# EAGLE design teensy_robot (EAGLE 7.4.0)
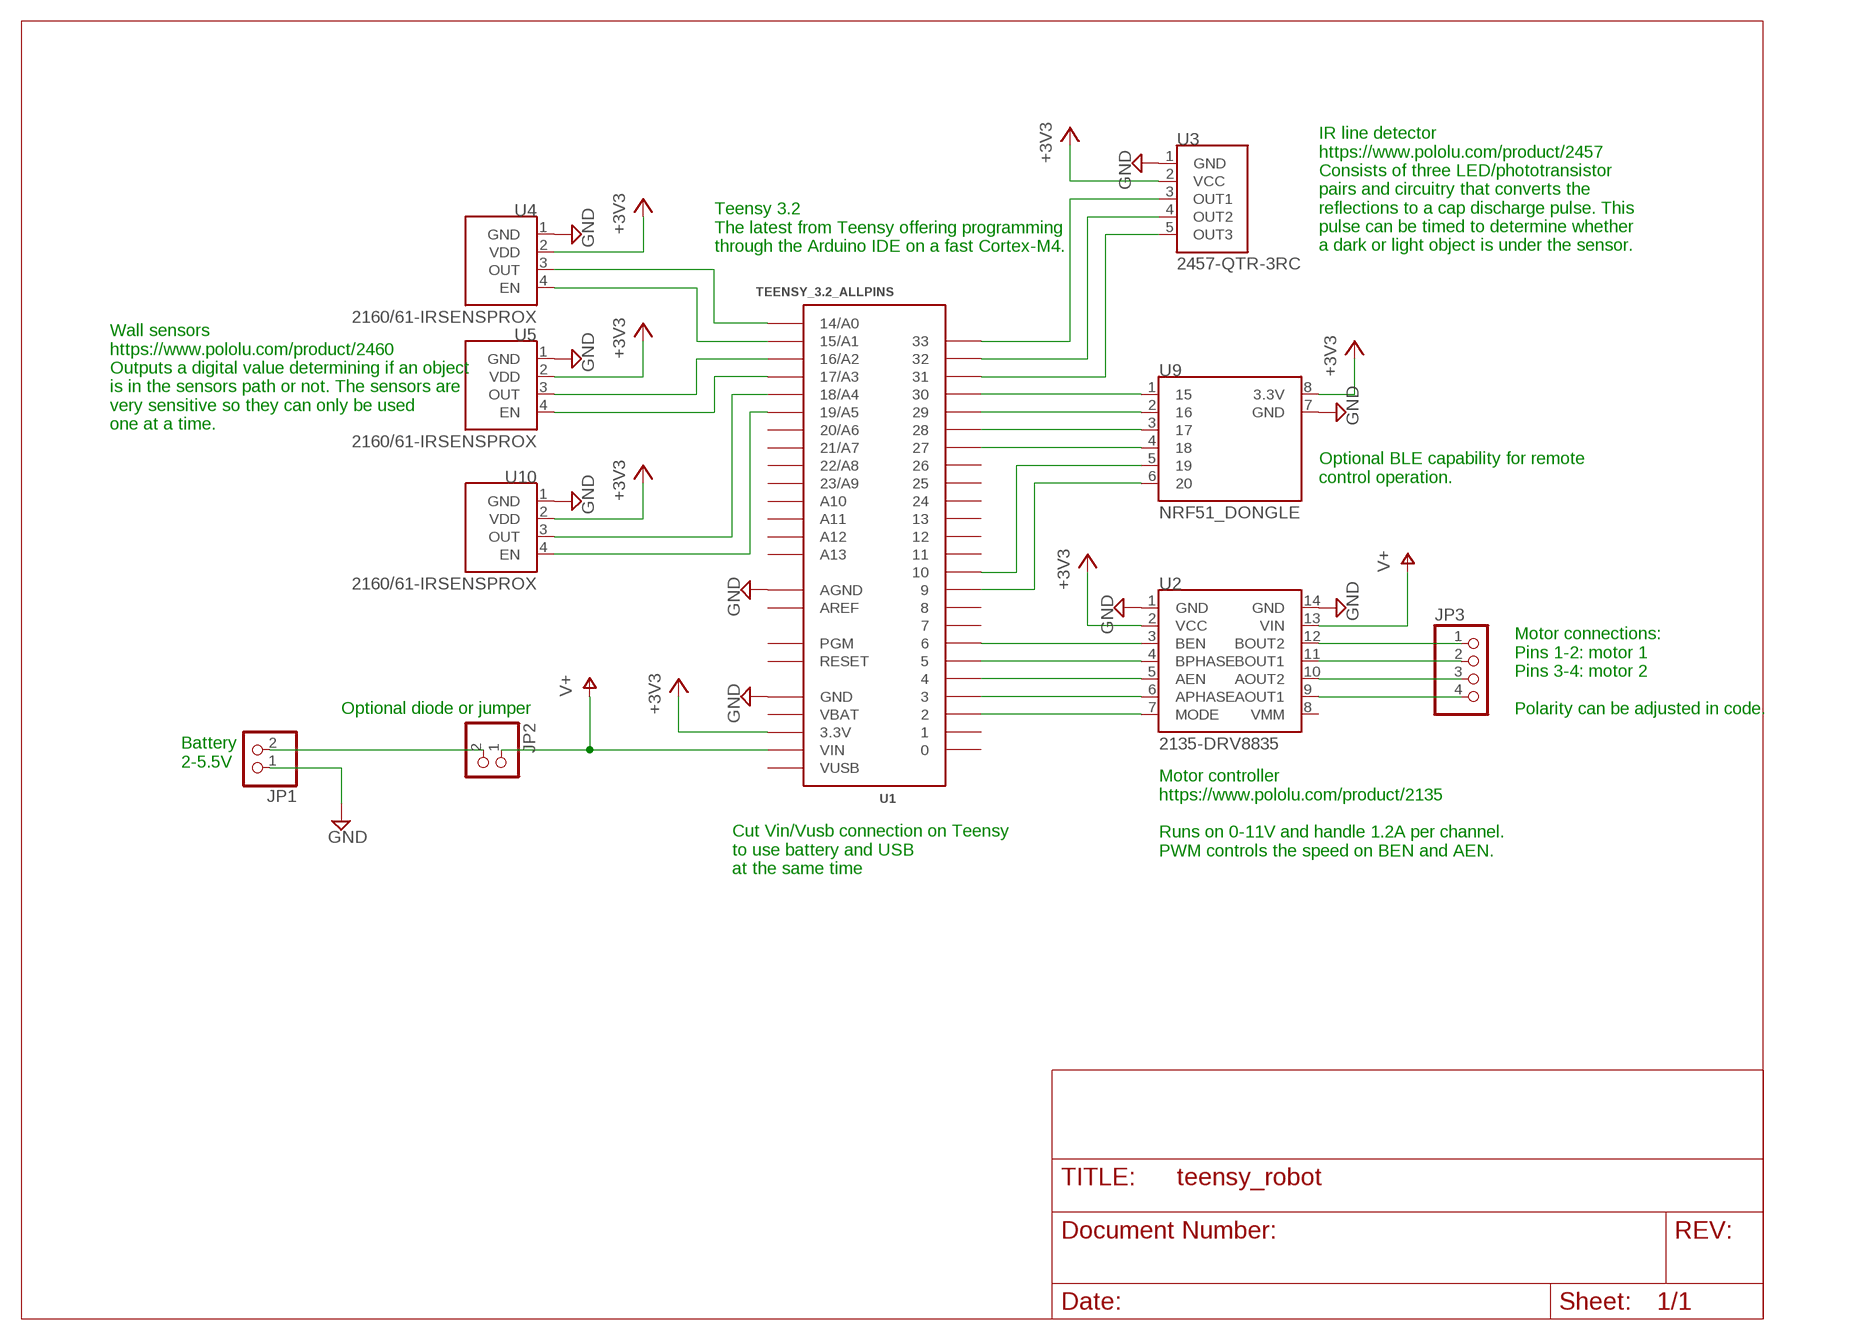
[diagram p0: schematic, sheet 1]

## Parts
JP1  PINHD-1X2  [1X02]
JP2  PINHD-1X2  [1X02]
JP3  PINHD-1X4  [1X04]
U1  TEENSY_3.2_ALLPINS  [TEENSY_3.0_ALLPINS]
U2  2135-DRV8835  [DIL14]
U3  2457-QTR-3RC  [QTR-3RC]
U4  2160/61-IRSENSPROX  [IRSENSPROX]
U5  2160/61-IRSENSPROX  [IRSENSPROX]
U9  NRF51_DONGLE  [NRF51_DONGLE_PACK]
U10  2160/61-IRSENSPROX  [IRSENSPROX]

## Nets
+3V3: U1.3.3V U1.3.3V1(3.3V) U1.3.3V2(3.3V) U2.2(VCC) U3.2(VCC) U4.2(VDD) U5.2(VDD) U9.8(3.3V) U10.2(VDD)
GND: JP1.1 U1.AGND U1.GND U1.GND1(GND) U1.GND2(GND) U2.1(GND) U2.14(GND) U3.1(GND) U4.1(GND) U5.1(GND) U9.7(GND) U10.1(GND)
N$1: JP1.2 JP2.2
N$2: U1.17/A3 U5.4(EN)
N$3: U1.6 U2.3(BEN)
N$4: U1.19/A5 U10.4(EN)
N$5: U1.9 U9.6
N$6: U1.10 U9.5
N$7: U1.16/A2 U5.3(OUT)
N$8: U1.14/A0 U4.3(OUT)
N$9: U1.15/A1 U4.4(EN)
N$10: U1.5 U2.4(BPHASE)
N$11: U1.4 U2.5(AEN)
N$12: U1.3 U2.6(APHASE)
N$13: U1.2 U2.7(MODE)
N$14: U1.31 U3.5(OUT3)
N$15: U1.32 U3.4(OUT2)
N$16: JP3.1 U2.12(BOUT2)
N$17: JP3.2 U2.11(BOUT1)
N$18: JP3.3 U2.10(AOUT2)
N$19: JP3.4 U2.9(AOUT1)
N$20: U1.33 U3.3(OUT1)
N$21: U1.27 U9.4
N$22: U1.28 U9.3
N$23: U1.29 U9.2
N$24: U1.30 U9.1
N$25: U1.18/A4 U10.3(OUT)
V+: JP2.1 U1.VIN U2.13(VIN)
Unconnected: U1.0 U1.1 U1.7 U1.8 U1.11 U1.12 U1.13 U1.20/A6 U1.21/A7 U1.22/A8 U1.23/A9 U1.24 U1.25 U1.26 U1.A10 U1.A11 U1.A12 U1.A13 U1.PGM U1.RESET U2.8(VMM)

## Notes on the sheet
- Teensy 3.2
  The latest from Teensy offering programming
  through the Arduino IDE on a fast Cortex-M4.
- IR line detector
  https://www.pololu.com/product/2457
  Consists of three LED/phototransistor
  pairs and circuitry that converts the
  reflections to a cap discharge pulse. This
  pulse can be timed to determine whether
  a dark or light object is under the sensor.
- Wall sensors
  https://www.pololu.com/product/2460
  Outputs a digital value determining if an object
  is in the sensors path or not. The sensors are
  very sensitive so they can only be used
  one at a time.
- Optional BLE capability for remote
  control operation.
- Optional diode or jumper
- Motor connections:
  Pins 1-2: motor 1
  Pins 3-4: motor 2
  
  Polarity can be adjusted in code.
- Battery
  2-5.5V
- Motor controller
  https://www.pololu.com/product/2135
  
  Runs on 0-11V and handle 1.2A per channel.
  PWM controls the speed on BEN and AEN.
- Cut Vin/Vusb connection on Teensy
  to use battery and USB
  at the same time

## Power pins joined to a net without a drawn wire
AREF: U1.AREF
VBAT: U1.VBAT
VUSB: U1.VUSB

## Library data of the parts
JP1 JP2 = pinhead:PINHD-1X2: PIN HEADER
JP3 = pinhead:PINHD-1X4: PIN HEADER
U1 = Teensy3.0:TEENSY_3.2_ALLPINS: Teensy 3.0 with all pin holes and optional SMD-mount unshrouded header on bottom of Teensy 3.0. For more basic versions, see 'Basic', '+4' and 'AllAnalogPins'. Requires the installation of a un-shrouded SMD header on the underside of the Teensy 3.0
U2 = pololu:2135-DRV8835: https://www.pololu.com/product/2135 This tiny breakout board for TI’s DRV8835 dual motor driver can deliver 1.2 A per channel continuously (1.5 A peak) to a pair of DC motors, and it supports two possible control interfaces for added flexibility of use: IN/IN and PHASE/ENABLE. With an operating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
U3 = pololu:2457-QTR-3RC: https://www.pololu.com/product/2457 This compact module packs three IR LED/phototransistor pairs onto a 1.25″ × 0.3″ board. The sensors are mounted on a 0.375″ pitch, allowing this array to be used as a minimal detector for a line-following robot. Each sensor provides a separate digital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
U4 U5 U10 = pololu:2160/61-IRSENSPROX: https://www.pololu.com/product/2460 This module features a fixed-gain, 38 kHz modulated IR sensor and a corresponding IR LED with oscillator circuit to make a tiny proximity sensor. This low-brightness version draws an average of 8 mA and has a typical sensing range up to approximately 12 inches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
U9 = pololu:NRF51_DONGLE: https://www.nordicsemi.com/eng/Products/nRF51-Dongle The nRF51 Dongle is a low-cost, versatile USB development dongle for Bluetooth® Smart, ANT and 2.4GHz proprietary applications using the nRF51 Series SoC. The dongle supports development for nRF51822 and nRF51422 SoCs.

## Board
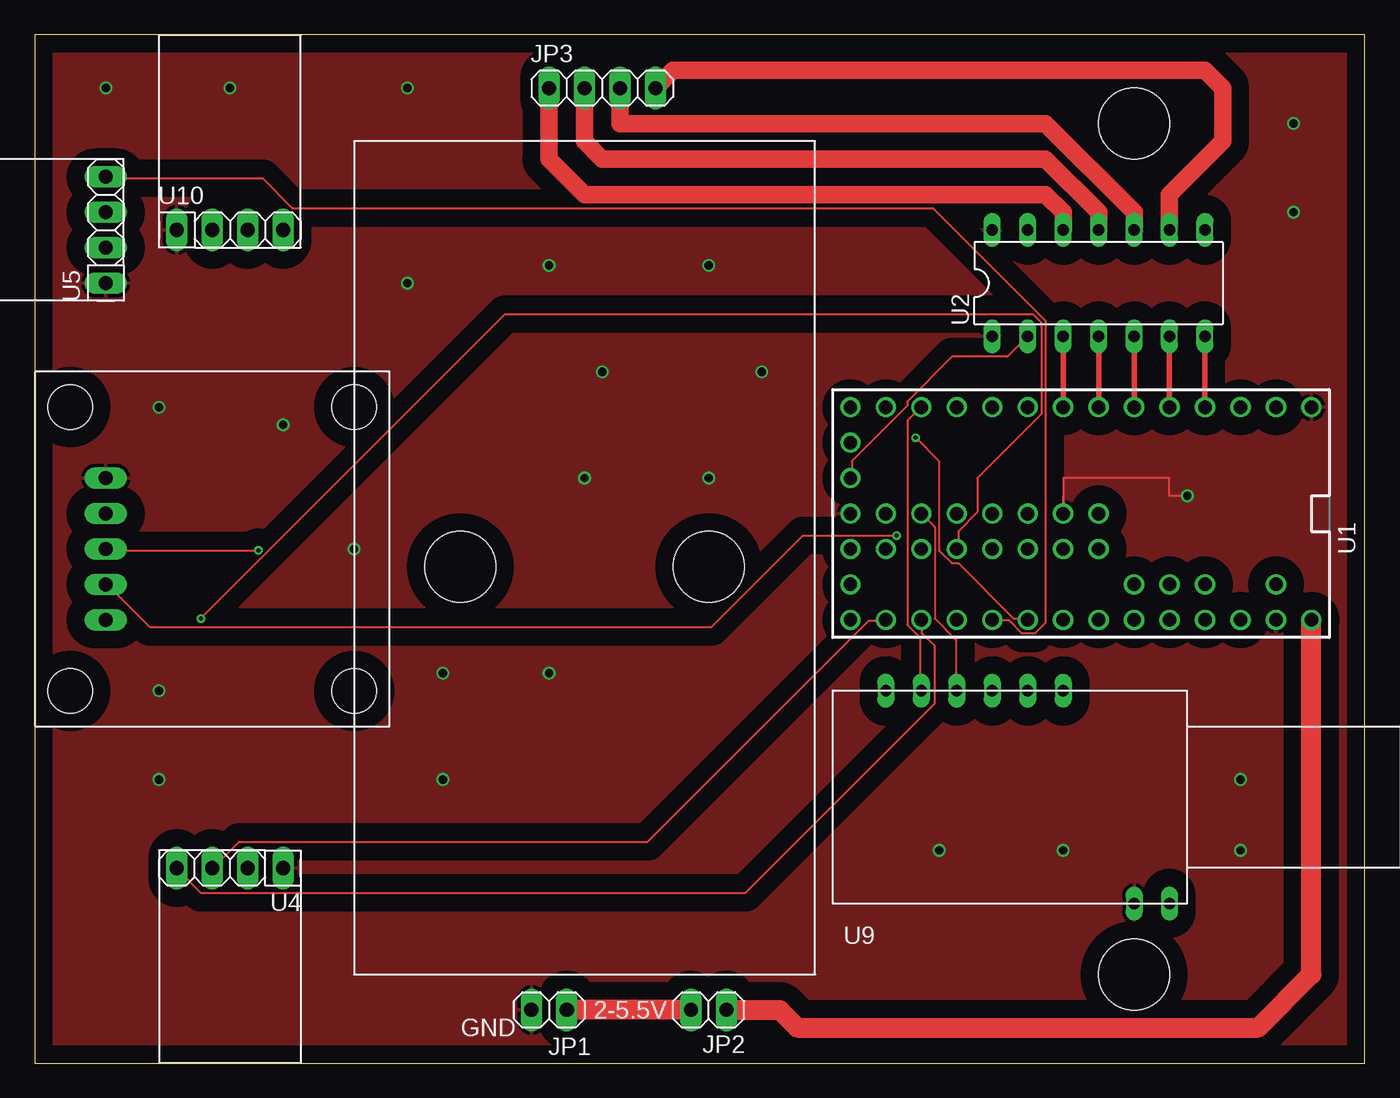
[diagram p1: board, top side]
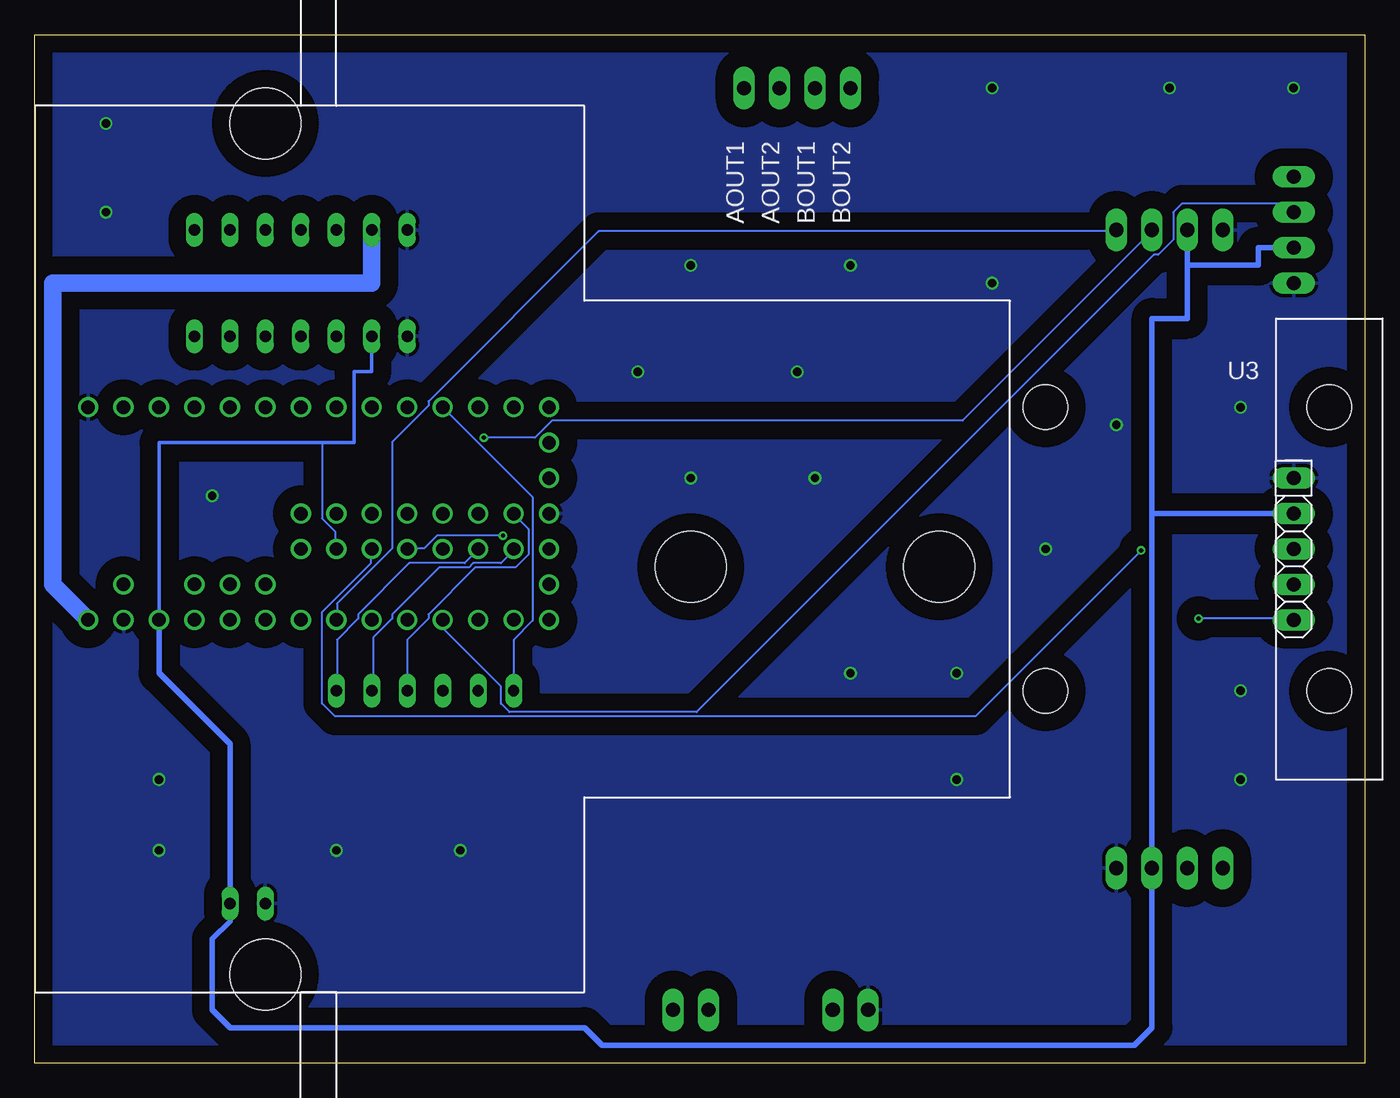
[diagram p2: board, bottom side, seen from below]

Size 95.25 x 73.66 mm. Coordinates in mm from the lower left corner, seen from the top.
Outline: 0,0 95.25,0 95.25,73.66 0,73.66 0,0
Copper layers (1*16): Top 0.035mm / dielectric 1.6mm / Bottom 0.035mm
Design rules "Elecrow_2-layer_PCB_eagle_rule": minimum track width 6mil, minimum drill 12mil, track to track 6mil, track to pad 6mil, pad to pad 6mil, via to via 8mil, smd to smd 0mil, copper to edge 20mil, drill to drill 10mil, minimum pad ring 6mil, minimum via ring 6mil, stop-mask expansion 0mil, vias tented up to drill 100mil, thermal gap 10mil

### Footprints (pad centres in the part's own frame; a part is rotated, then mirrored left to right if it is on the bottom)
1X02 = drill 1.016 long: 1 -1.27,0; 2 1.27,0
1X04 = drill 1.016 long: 1 -3.81,0; 2 -1.27,0; 3 1.27,0; 4 3.81,0
TEENSY_3.0_ALLPINS = drill 0.965: 0 -7.62,13.97; 1 -7.62,11.43; 2 -7.62,8.89; 3 -7.62,6.35; 3.3V 7.62,11.43; 3.3V1 -2.54,-16.51; 3.3V2 2.54,-1.27; 4 -7.62,3.81; 5 -7.62,1.27; 6 -7.62,-1.27; 7 -7.62,-3.81; 8 -7.62,-6.35; 9 -7.62,-8.89; 10 -7.62,-11.43; 11 -7.62,-13.97; 12 -7.62,-16.51; 13 7.62,-16.51; 14/A0 7.62,-13.97; 15/A1 7.62,-11.43; 16/A2 7.62,-8.89; 17/A3 7.62,-6.35; 18/A4 7.62,-3.81; 19/A5 7.62,-1.27; 20/A6 7.62,1.27; 21/A7 7.62,3.81; 22/A8 7.62,6.35; 23/A9 7.62,8.89; 24 0,-3.81; 25 0,-6.35; 26 0,-8.89; 27 0,-11.43; 28 0,-13.97; 29 2.54,-13.97; 30 2.54,-11.43; 31 2.54,-8.89; 32 2.54,-6.35; 33 2.54,-3.81; A10 5.08,6.35; A11 5.08,3.81; A12 0,1.27; A13 2.54,1.27; AGND 7.62,13.97; AREF 5.08,8.89; GND -7.62,16.51; GND1 0,-16.51; GND2 0,-1.27; PGM 2.54,-16.51; RESET 5.08,-16.51; VBAT -5.08,-16.51; VIN 7.62,16.51; VUSB 5.08,13.97
DIL14 = drill 0.813 long: 1 -7.62,-3.81; 2 -5.08,-3.81; 3 -2.54,-3.81; 4 0,-3.81; 5 2.54,-3.81; 6 5.08,-3.81; 7 7.62,-3.81; 8 7.62,3.81; 9 5.08,3.81; 10 2.54,3.81; 11 0,3.81; 12 -2.54,3.81; 13 -5.08,3.81; 14 -7.62,3.81
QTR-3RC = drill 1.016 long: 1 -5.08,0; 2 -2.54,0; 3 0,0; 4 2.54,0; 5 5.08,0
IRSENSPROX = drill 1.016 long: 1 -3.81,0; 2 -1.27,0; 3 1.27,0; 4 3.81,0
NRF51_DONGLE_PACK = drill 0.813 long: 1 0,0; 2 2.54,0; 3 5.08,0; 4 7.62,0; 5 10.16,0; 6 12.7,0; 7 -5.08,15.24; 8 -7.62,15.24
2AA_BATTERYHOLDER = hole 5.08: 29.21,25.4; 29.21,7.62
TAMIYA_70168 = hole 5.08: 1.27,53.34; 62.23,53.34
TAMIYA_70144_BALL = hole 3.2: 0,0; 20.32,0; 0,20.32; 20.32,20.32

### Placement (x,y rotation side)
JP1  36.83,3.81 0 top
JP2  48.26,3.81 180 top
JP3  40.64,69.85 0 top
U1  74.93,39.37 270 top
U2  76.2,55.88 0 top
U3  5.08,36.83 270 bottom
U4  13.97,13.97 180 top
U5  5.08,59.69 90 top
U9  73.66,26.67 180 top
U10  13.97,59.69 0 top
U$6  [2AA_BATTERYHOLDER]  55.88,6.35 90 top
U$7  [TAMIYA_70168]  25.4,5.08 90 bottom
U$8  [TAMIYA_70144_BALL]  2.54,26.67 0 top

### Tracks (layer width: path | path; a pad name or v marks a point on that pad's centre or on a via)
+3V3
  Top 0.152: U2.2 69.65,50.6 65.68,50.6 62.48,47.4 62.48,47.09 58.52,43.13 58.52,41.91 U1.3.3V1
  Bottom 0.152: 74.68,44.45 74.68,39.01 73.76,38.1 73.76,36.88 U1.3.3V2
  Bottom 0.254: U2.2 71.12,49.53 72.39,49.53 72.39,44.45 74.68,44.45 86.36,44.45 U1.3.3V
  Bottom 0.406: U1.3.3V 86.36,27.94 81.28,22.86 U9.8 81.28,10.16 82.55,8.89 82.55,3.81 81.28,2.54 55.88,2.54 54.61,1.27 16.51,1.27 15.24,2.54 U4.2 15.24,39.37 | 15.24,39.37 U3.2 | 15.24,39.37 15.24,53.34 12.7,53.34 12.7,57.15 | 12.7,57.15 U10.2 | U5.2 7.62,58.42 7.62,57.15 12.7,57.15
GND  (via drill 0.6)
  Top 0.152: 73.66,40.64 U1.GND2 73.66,41.91 81.28,41.91 81.28,40.64 v82.55,40.64
  other vias: 5.08,69.85 13.97,69.85 26.67,69.85 26.67,55.88 36.83,57.15 48.26,57.15 52.07,49.53 40.64,49.53 39.37,41.91 48.26,41.91 36.83,27.94 29.21,27.94 22.86,36.83 17.78,45.72 8.89,46.99 8.89,26.67 8.89,20.32 29.21,20.32 64.77,15.24 73.66,15.24 90.17,67.31 90.17,60.96 86.36,20.32 86.36,15.24
  pour Bottom (isolate 1.27): 0,0 0,73.66 95.25,73.66 95.25,0
  pour Top (isolate 1.27): 0,0 0,73.66 95.25,73.66 95.25,0
N$1
  Top 1.422: JP2.2 JP1.2
N$2
  Top 0.152: U1.17/A3 68.58,31.7 69.8,31.7 70.71,30.79 71.63,30.79 72.39,31.55 72.39,53.19 64.31,61.27 18.44,61.27 16.31,63.4 5.18,63.4 U5.4
N$3
  Top 0.406: U1.6 U2.3
N$4
  Bottom 0.152: U1.19/A5 73.61,31.85 73.61,32.92 69.65,36.88 69.65,44.5 67.06,47.09 67.06,47.4 54.86,59.59 17.83,59.59 U10.4
N$5
  Bottom 0.152: U9.6 60.96,30.33 59.59,31.7 59.59,40.54 U1.9
N$6
  Top 0.152: U9.5 63.4,26.67 63.4,30.48 62.48,31.39 62.48,46.02 63.4,46.94 U1.10
N$7
  Bottom 0.152: U1.16/A2 65.99,31.7 65.99,31.09 61.87,26.98 61.87,25.76 61.27,25.15 47.85,25.15 15.09,57.91 14.78,57.91 13.72,58.98 13.72,60.96 13.11,61.57 5.79,61.57 5.18,60.96 U5.3
N$8
  Top 0.152: U1.14/A0 60.96,31.7 59.74,31.7 43.89,15.85 14.63,15.85 12.8,14.02 U4.3
N$9
  Top 0.152: U1.15/A1 63.55,31.7 63.55,30.79 64.47,29.87 64.47,25.76 50.9,12.19 11.89,12.19 10.21,13.87 U4.4
N$10
  Top 0.406: U1.5 U2.4
N$11
  Top 0.406: U1.4 U2.5
N$12
  Top 0.406: U1.3 U2.6
N$13
  Top 0.406: U1.2 U2.7
N$14  (via drill 0.3)
  Top 0.152: v11.89,31.85 33.68,53.65 71.48,53.65 72.08,53.03 72.08,46.48 67.51,41.91 67.51,39.47 66.14,38.1 66.14,36.88 U1.31
  Bottom 0.152: v11.89,31.85 5.18,31.85 U3.5
N$15  (via drill 0.3)
  Top 0.152: v61.72,37.8 55.02,37.8 48.46,31.24 8.23,31.24 5.18,34.29 U3.4
  Bottom 0.152: v61.72,37.8 66.45,37.8 67.36,36.88 68.58,36.88 U1.32
N$16
  Top 1.27: JP3.1 36.83,64.77 39.37,62.23 72.39,62.23 73.66,60.96 U2.12
N$17
  Top 1.27: U2.11 76.2,60.96 72.39,64.77 40.64,64.77 39.37,66.04 JP3.2
N$18
  Top 1.27: U2.10 78.74,60.96 72.39,67.31 41.91,67.31 JP3.3
N$19
  Top 1.27: U2.9 81.28,62.23 85.09,66.04 85.09,69.85 83.82,71.12 45.72,71.12 JP3.4
N$20  (via drill 0.3)
  Top 0.152: v16,36.73 5.18,36.73 U3.3
  Bottom 0.152: v16,36.73 27.89,24.84 73.76,24.84 74.68,25.76 74.68,32.31 71.17,35.81 71.17,36.73 U1.33
N$21
  Top 0.152: U1.27 64.47,38.41 64.47,31.85 65.99,30.33 65.99,26.67 U9.4
N$22
  Bottom 0.152: U9.3 68.58,30.33 67.06,31.85 67.06,32.16 63.7,35.51 60.81,35.51 59.89,36.42 59.89,38.25 60.96,39.32 U1.28
N$23
  Bottom 0.152: U9.2 71.02,26.67 71.02,30.48 69.65,31.85 69.65,32.16 66.29,35.51 64.16,35.51 63.86,35.81 61.87,35.81 60.96,36.73 U1.29
N$24
  Bottom 0.152: U9.1 73.61,26.67 73.61,30.33 72.08,31.85 72.08,32.16 68.43,35.81 64.47,35.81 63.55,36.73 U1.30
N$25  (via drill 0.3)
  Top 0.152: v63.09,44.81 64.77,43.13 64.77,36.73 65.68,35.81 66.14,35.81 70.1,31.85 71.02,31.85 U1.18/A4
  Bottom 0.152: v63.09,44.81 59.44,44.81 58.22,46.02 28.8,46.02 15.24,59.59 U10.3
V+
  Top 1.422: JP2.1 53.34,3.81 54.61,2.54 87.63,2.54 91.44,6.35 U1.VIN
  Bottom 1.27: U2.13 71.12,55.88 93.98,55.88 93.98,34.29 U1.VIN

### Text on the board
tPlace: 2-5.5V | GND
bPlace: BOUT2 | BOUT1 | AOUT2 | AOUT1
